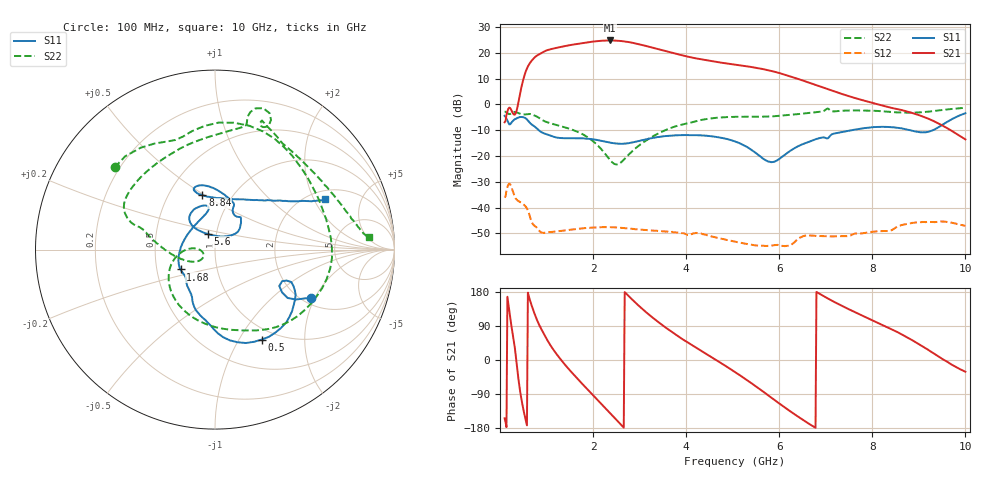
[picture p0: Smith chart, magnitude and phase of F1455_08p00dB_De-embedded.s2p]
! Integrated Device Technology
! Corporate Headquarters
! 6024 Silver Creek Valley Road
! San Jose, CA 95138  USA
! Phone:  1-408-284-8200
! Toll Free:  1-800-223-1366
! Webpage:  http://www.idt.com/
! Timing and RF Division
! 515 Groton Road, Suite 102
! Westford, MA 01886-6024
! Device:  F1455
! Description: 6-bit 0.5 dB Transmit Variable Gain Amplifier
! Frequency:  1400.0 -  2300.00 MHz
! Package:  6x6 mm Thin QFN Plastic Package: 28 pin
! State:  16
! Atten State:  8.0 dB
! Voltage:  +5.00 Volts
! Current:  217.680 mA
! Data:  The device was measured on a the F1455 evaluation board which has
!  individual transmission lines to the RF pins.  Data was collected
!  using a calibrated network analyzer.  The evaluation board was
!  de-embedded using a TRL calibration technique.
!  The reference plane is the edge of the package pin.
!  Pin  1 = CSb
!  Pin  2 = DATA
!  Pin  3 = CLK
!  Pin  4 = RSET
!  Pin  5 = GND
!  Pin  6 = RFIN  = Port 1
!  Pin  7 = GND
!  Pin  8 = NC
!  Pin  9 = NC
!  Pin 10 = NC
!  Pin 11 = NC
!  Pin 12 = NC
!  Pin 13 = NC
!  Pin 14 = /STBY
!  Pin 15 = GND
!  Pin 16 = RFOUT  = Port 2
!  Pin 17 = GND
!  Pin 18 = NC
!  Pin 19 = NC
!  Pin 20 = NC
!  Pin 21 = GND
!  Pin 22 = NC
!  Pin 23 = GND
!  Pin 24 = NC
!  Pin 25 = NC
!  Pin 26 = NC
!  Pin 27 = GND
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# GHz S dB R 50
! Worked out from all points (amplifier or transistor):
!   496 points, 100 MHz to 10 GHz, reference 50 ohm
!   highest |S21| = 24.8 dB at 2.36 GHz (marker M1)
!   |S21| within 3 dB of that: 1.181 GHz to 3.322 GHz (2.14 GHz wide, 95.1 % of centre)
!   unconditionally stable (mu >= 1): start of sweep to end of sweep
!   at 1.74 GHz: K = 7.26, MAG = 24.3 dB, |S12| = -48.0 dB
!   at 5.06 GHz: K = 24.89, MAG = 17.3 dB, |S12| = -53.2 dB
!   at 10 GHz: K = 74.46, MAG = -5.0 dB, |S12| = -47.0 dB
!   S11 on the Smith chart (normalised r, x): 100 MHz: 2.22, -1.87; 500 MHz: 0.85, -1.25; 1.68 GHz: 0.66, -0.15; 5.6 GHz: 0.91, +0.16; 8.84 GHz: 0.73, +0.49; 10 GHz: 2.40, +2.46
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0.1  -4.44 -26.8  -6.90 -153.8  -36.09 44.1  -2.81 140.7
0.38  -5.20 -38.7  -0.69 -32.7  -37.23 -110.8  -3.24 56.2
0.5  -4.96 -62.6  9.57 -128.6  -38.66 -148.6  -3.83 27.8
0.68  -7.73 -95.4  16.91 144.1  -45.41 151.1  -3.83 -14.7
0.82  -9.76 -112.0  19.20 98.6  -48.45 134.3  -4.97 -47.7
0.96  -11.30 -120.8  20.59 65.2  -49.74 123.4  -6.51 -72.3
1.3  -13.02 -137.6  22.26 2.3  -49.03 83.5  -8.38 -116.6
1.68  -13.09 -150.0  23.52 -51.4  -48.20 49.6  -10.70 -152.0
1.76  -13.10 -153.0  23.75 -61.9  -48.03 43.5  -11.39 -158.2
2.06  -13.66 -168.3  24.47 -100.6  -47.64 22.7  -15.17 -177.8
2.36  -14.75 167.3  24.79 -139.7  -47.54 3.6  -21.39 -179.6
2.54  -15.22 148.3  24.68 -163.0  -47.74 -7.0  -23.13 -155.6
2.74  -15.04 127.7  24.24 171.8  -48.03 -17.2  -19.94 -144.3
3.06  -13.84 105.3  23.01 134.6  -48.56 -31.1  -14.97 -160.4
3.4  -12.63 98.7  21.41 100.3  -49.03 -43.7  -11.28 -179.1
4.1  -11.89 111.6  18.25 41.1  -50.30 -65.4  -7.04 163.4
5.06  -14.38 133.4  15.42 -32.6  -53.19 -102.4  -4.80 148.3
5.6  -20.23 115.3  13.87 -78.5  -54.79 -108.3  -4.75 127.0
6.7  -14.05 44.2  8.07 -172.9  -50.80 -140.9  -3.18 78.3
8.36  -8.75 107.8  -1.10 84.0  -48.99 164.5  -2.82 62.3
8.84  -10.13 103.1  -3.22 53.3  -45.98 147.3  -3.19 44.0
10  -3.42 24.5  -13.55 -31.0  -47.02 76.8  -1.30 4.6
